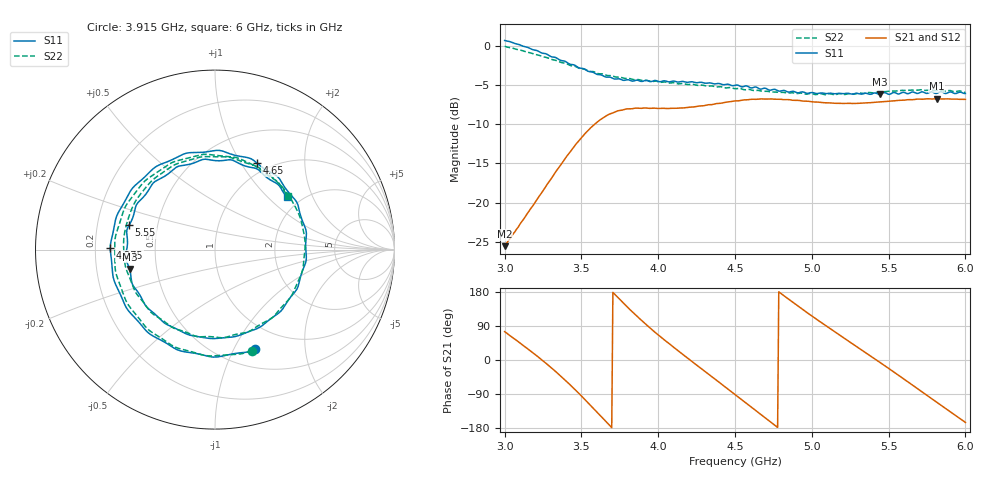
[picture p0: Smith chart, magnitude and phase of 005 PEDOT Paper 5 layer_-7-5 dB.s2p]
!  04/11/2025  19:13:25
! Ref Plane: 0.000 mm
# MHZ S MA R  50
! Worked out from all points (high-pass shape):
!   401 points, 3 GHz to 6 GHz, reference 50 ohm
!   highest |S21| = -6.77 dB at 5.812 GHz (marker M1); lowest = -25.5 dB at 3 GHz (marker M2)
!   |S21| within 3 dB of the highest: 3.602 GHz to end of sweep
!   lowest |S11| = -6.2 dB at 5.445 GHz (marker M3), VSWR 2.91, Z = 17.4 - j4.93 ohm
!   |S11| at or under -10 dB: nowhere
!   |S22| runs from -6.3 to -0.1 dB; largest |S21 - S12| = 0.0086
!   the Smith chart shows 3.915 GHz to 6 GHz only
!   S11 on the Smith chart (normalised r, x): 3.915 GHz: 0.70, -1.22; 4.275 GHz: 0.26, +0.01; 4.65 GHz: 0.86, +1.17; 5.55 GHz: 0.34, +0.12; 6 GHz: 1.70, +1.31
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3000  1.077 -113.3  0.05291 74.8  0.05339 75.7  0.9892 -116.9
3142.5  0.9779 -146.9  0.08369 31.9  0.08399 32.8  0.9101 -150.2
3262.5  0.8891 -177.7  0.1244 -6.2  0.1244 -5.6  0.8438 178.7
3390  0.7963 144.6  0.189 -51.4  0.1896 -51.0  0.7725 139.9
3502.5  0.7163 104.1  0.261 -95.8  0.2614 -95.5  0.7101 99.1
3592.5  0.6613 67.8  0.3194 -133.6  0.321 -133.5  0.6741 62.9
3705  0.6177 18.2  0.3725 178.4  0.3747 178.8  0.6391 14.1
3802.5  0.6059 -24.4  0.3957 138.2  0.3974 139.2  0.6171 -27.2
3915  0.5994 -68.1  0.4006 95.7  0.4022 96.8  0.5989 -69.9
4005  0.589 -98.2  0.3978 64.8  0.3979 65.5  0.5863 -100.1
4155  0.5907 -145.2  0.4006 16.3  0.4039 16.9  0.5729 -147.4
4275  0.5836 179.1  0.4126 -21.2  0.4145 -20.4  0.5595 176.1
4500  0.5585 110.4  0.444 -91.1  0.4466 -90.4  0.5313 106.0
4650  0.5364 64.4  0.4558 -137.9  0.4569 -137.6  0.5186 57.1
4815  0.5183 11.7  0.4526 170.7  0.453 171.4  0.5034 3.8
5002.5  0.5021 -43.2  0.4383 115.6  0.4379 116.2  0.4941 -52.0
5220  0.4959 -104.4  0.4286 55.0  0.4289 55.5  0.4886 -112.1
5445  0.4884 -167.2  0.4376 -6.8  0.4389 -6.0  0.5081 -171.6
5505  0.4887 176.0  0.4424 -23.5  0.4442 -22.6  0.512 172.0
5550  0.4973 164.1  0.4462 -36.2  0.4478 -35.2  0.5135 159.6
5812.5  0.4955 87.1  0.4589 -111.4  0.4614 -110.6  0.5174 86.8
6000  0.4948 36.0  0.4544 -164.7  0.4558 -164.1  0.5041 36.0
